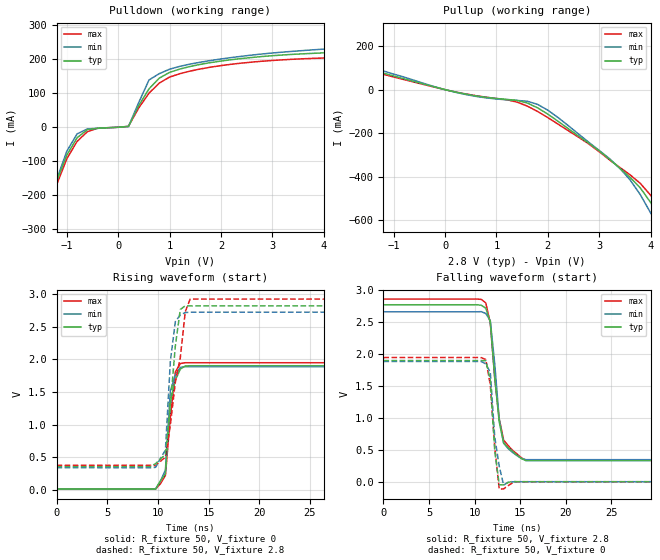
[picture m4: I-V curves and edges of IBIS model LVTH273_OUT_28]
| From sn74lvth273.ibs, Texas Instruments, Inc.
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|   Model LVTH273_OUT_28
[Model]   LVTH273_OUT_28
Model_type  Output
Polarity   Non-Inverting
Vmeas = 1.5v
Cref = 50pf
Rref = 500
Vref = 0V
| variable   typ   min   max
C_comp   7p   NA   NA
[Temperature Range]   40   -25   100
| Ambient temperature   25   -40   85
[Voltage range]   2.8   2.7   2.9
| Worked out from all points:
|   slope of the pulldown table from 0 to 0.42 V, typ, clamps not added: 6.12 ohm
|   slope of the pullup table from 0 to 0.42 V, typ, clamps not added: 19.7 ohm
|   rising waveform, R_fixture 50, V_fixture 0: 20-80 % time 688ps typ, 455ps min, 708ps max; typ from 0.01 V to 1.9 V
|   falling waveform, R_fixture 50, V_fixture 2.8: 20-80 % time 1.03ns typ, 961ps min, 1.11ns max; typ from 2.78 V to 0.34 V
|   rising waveform, R_fixture 50, V_fixture 2.8: 20-80 % time 885ps typ, 636ps min, 1.36ns max; typ from 0.357 V to 2.82 V
|   falling waveform, R_fixture 50, V_fixture 0: 20-80 % time 552ps typ, 735ps min, 656ps max; typ from 1.91 V to 0.011 V
[Pulldown]
|   Voltage   I(typ)   I(min)   I(max)
-5V       -3.149A    -3.526A    -2.821A
-1.6V     -381.5mA   -396.9mA   -415.3mA
-1.4V     -260.7mA   -265.5mA   -278.1mA
-1V       -82.03mA   -70.61mA   -92.59mA
-800mV    -31.23mA   -19.8mA    -41.76mA
-400mV    -3.148mA   -3.5mA     -3.397mA
200mV     2.075mA    1.837mA    2.435mA
600mV     112.4mA    138.4mA    99.65mA
1.2V      170.4mA    178.3mA    156.8mA
3V        209.5mA    217.4mA    195.5mA
8.2V      247.6mA    293.9mA    223.8mA
10V       269.2mA    340.7mA    239.3mA
[Pullup]
|   Voltage   I(typ)   I(min)   I(max)
-5V       244.6mA    283.6mA    221.7mA
-3.6V     230.7mA    252mA      212.3mA
-3.4V     230.7mA    250.2mA    186.4mA
-3.2V     189.8mA    211.3mA    178.1mA
0V        91.21uA    94.36uA    63.56uA
1.4V      -49.28mA   -49.51mA   -57.08mA
1.8V      -83.42mA   -67.56mA   -100.1mA
3.4V      -361.2mA   -361.9mA   -357.5mA
3.8V      -452.3mA   -483.3mA   -431.3mA
4.2V      -594.6mA   -636.5mA   -561.4mA
4.4V      -662.9mA   -720.4mA   -634.3mA
10V       -2.817A    -3.081A    -2.568A
[Ramp]
| variable   typ   min   max
dV/dt_r  1.164E+00/7.090E-10  1.158E+00/6.710E-10  1.200E+00/7.120E-10
dV/dt_f  1.458E+00/7.760E-10  1.390E+00/6.780E-10  1.500E+00/8.450E-10
R_load = 50
[Rising Waveform]
R_fixture = 50
V_fixture = 0
V_fixture_min = 0
V_fixture_max = 0
C_fixture = 0pf
L_fixture = 0nH
|   Time   V(typ)   V(min)   V(max)
0s        10.06mV    10.66mV    10.15mV
9.766ns   10.07mV    12.89mV    10.85mV
10.25ns   138.9mV    131.9mV    93.08mV
10.74ns   244.7mV    304.9mV    219.4mV
11.23ns   1.345V     1.518V     1.118V
11.72ns   1.682V     1.762V     1.807V
12.21ns   1.853V     1.878V     1.938V
12.7ns    1.9V       1.89V      1.95V
13.18ns   1.904V     1.89V      1.95V
49.71ns   1.904V     1.89V      1.95V
[Falling Waveform]
R_fixture = 50
V_fixture = 2.8
V_fixture_min = 2.7
V_fixture_max = 2.9
C_fixture = 0pf
L_fixture = 0nH
|   Time   V(typ)   V(min)   V(max)
0s        2.777V     2.667V     2.866V
10.25ns   2.777V     2.667V     2.866V
11.23ns   2.722V     2.64V      2.805V
11.72ns   2.509V     2.527V     2.489V
12.21ns   1.638V     1.85V      1.628V
12.7ns    943mV      982.2mV    993.1mV
13.18ns   620.4mV    613.7mV    661.5mV
14.16ns   485.4mV    468.8mV    502.8mV
15.63ns   340.1mV    355.1mV    347.8mV
49.71ns   340.1mV    355.1mV    347.8mV
[Rising Waveform]
R_fixture = 50
V_fixture = 2.8
V_fixture_min = 2.7
V_fixture_max = 2.9
C_fixture = 0pf
L_fixture = 0nH
|   Time   V(typ)   V(min)   V(max)
0s        357mV      339.9mV    375.5mV
9.277ns   357mV      338.8mV    375.5mV
9.766ns   401.4mV    344.5mV    370.4mV
10.74ns   537.6mV    608.4mV    500.8mV
11.23ns   1.297V     1.977V     998.1mV
11.72ns   2.208V     2.581V     1.65V
12.21ns   2.768V     2.685V     2.03V
12.7ns    2.823V     2.719V     2.733V
13.18ns   2.823V     2.726V     2.927V
49.71ns   2.823V     2.726V     2.927V
[Falling Waveform]
R_fixture = 50
V_fixture = 0
V_fixture_min = 0
V_fixture_max = 0
C_fixture = 0pf
L_fixture = 0nH
|   Time   V(typ)   V(min)   V(max)
0s        1.905V     1.89V      1.952V
10.74ns   1.905V     1.89V      1.95V
11.23ns   1.902V     1.852V     1.921V
11.72ns   1.606V     1.724V     1.521V
12.21ns   495.5mV    707.1mV    550.5mV
12.7ns    -36.58mV   252.8mV    -105.7mV
13.18ns   -38.42mV   -42.8mV    -101mV
13.67ns   -1.118mV   1.273mV    -51.35mV
14.65ns   10.73mV    10.68mV    10.57mV
49.71ns   10.73mV    10.67mV    10.57mV
